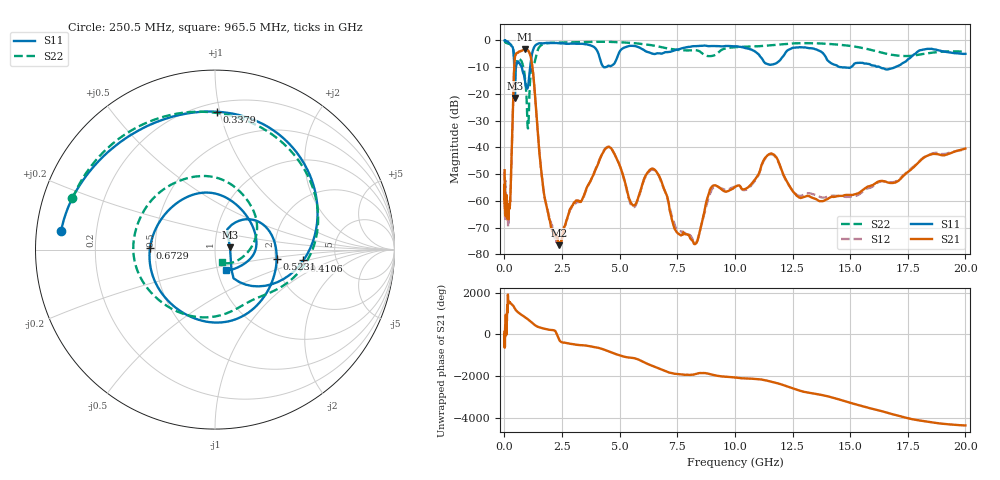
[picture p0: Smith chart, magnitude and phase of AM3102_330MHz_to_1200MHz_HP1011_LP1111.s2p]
! Date/Time: Tue, Sep 11, 2018 5:20 PM
! Network Analyzer: Agilent Technologies E8362B Rev: A.07.50.63
! Sweep from 0.010 to 20.000 GHz, 1601 Points, Sweep Type: LOG
! Power Supply: 4.949 V, 0.001 A
# Hz S DB R 50
!freq MagS11 AngS11 MagS21 AngS21 MagS12 AngS12 MagS22 AngS22
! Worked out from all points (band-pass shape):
!   1601 points, 10 MHz to 20 GHz, reference 50 ohm
!   highest |S21| = -3.28 dB at 916.3 MHz (marker M1); lowest = -76.7 dB at 2.381 GHz (marker M2)
!   |S21| within 3 dB of the highest: 457.6 MHz to 1.146 GHz (688.7 MHz wide, 85.9 % of centre)
!   lowest |S11| = -21.5 dB at 455.8 MHz (marker M3), VSWR 1.18, Z = 59 + j1.45 ohm
!   |S11| at or under -10 dB: 753.8 MHz to 1.118 GHz (364.4 MHz wide, 38.9 % of centre); 14.62 GHz to 15.03 GHz (412.9 MHz wide, 2.79 % of centre); 16.29 GHz to 16.95 GHz (658.9 MHz wide, 3.96 % of centre)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
!   |S22| runs from -32.9 to -0.2 dB; largest |S21 - S12| = 0.0093
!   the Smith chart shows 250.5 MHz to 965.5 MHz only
!   S11 on the Smith chart (normalised r, x): 250.5 MHz: 0.07, +0.06; 337.9 MHz: 0.26, +0.98; 410.6 MHz: 2.88, -0.46; 523.1 MHz: 2.03, -0.24; 672.9 MHz: 0.47, +0.01; 965.5 MHz: 1.10, -0.25
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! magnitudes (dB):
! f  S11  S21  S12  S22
! 10 MHz  0.0  -48.6  -49.1  -0.2
! 35.55 MHz  0.0  -64.1  -63.5  -0.5
! 126.4 MHz  -0.4  -64.0  -64.5  -1.1
! 250.5 MHz  -1.3  -59.9  -60.3  -1.5
! 337.9 MHz  -2.3  -36.0  -36.0  -2.3
! 410.6 MHz  -6.1  -13.6  -13.6  -5.1
! 447.2 MHz  -20.8  -7.1  -7.1  -8.6
! 455.8 MHz  -21.5  -6.4  -6.5  -9.1
! 523.1 MHz  -9.2  -4.8  -4.9  -7.8
! 672.9 MHz  -8.8  -4.1  -4.2  -7.1
! 916.3 MHz  -16.5  -3.3  -3.4  -15.9
! 965.5 MHz  -17.8  -3.4  -3.5  -22.0
! 1.224 GHz  -4.1  -10.5  -10.5  -8.6
! 1.59 GHz  -1.1  -48.0  -48.1  -1.8
! 2.381 GHz  -1.1  -76.7  -76.7  -0.8
! 4.457 GHz  -9.8  -40.0  -39.8  -0.5
! 5.652 GHz  -2.1  -61.6  -62.2  -1.0
! 6.518 GHz  -5.1  -48.3  -48.6  -2.0
! 8.149 GHz  -2.2  -74.8  -74.0  -3.7
! 11.47 GHz  -9.0  -42.6  -42.8  -1.9
! 13.87 GHz  -5.3  -59.9  -58.8  -1.2
! 20 GHz  -5.0  -40.4  -40.9  -4.1
